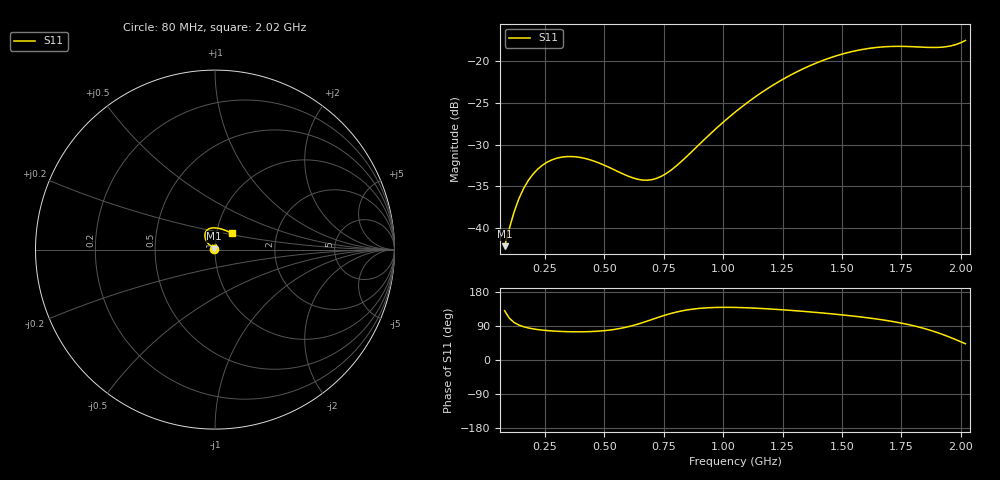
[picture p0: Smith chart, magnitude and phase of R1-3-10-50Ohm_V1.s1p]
!version-1
!date-08.2020
!Series
#	GHZ S RI R 50.0
!	FREQ.GHZ	S11RE	S11IM
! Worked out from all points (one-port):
!   98 points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, 80 MHz to 2.02 GHz, reference 50 ohm
!   lowest |S11| = -42.1 dB at 80 MHz (marker M1), VSWR 1.02, Z = 49.5 + j0.593 ohm
!   |S11| at or under -10 dB: start of sweep to end of sweep
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0.08  -0.00505 0.00599
0.12  -0.00197 0.0124
0.14  -0.000589 0.015
0.16  0.000676 0.0173
0.18  0.00183 0.0192
0.22  0.0038 0.0223
0.26  0.00532 0.0243
0.3  0.00639 0.0254
0.34  0.00701 0.0259
0.38  0.00719 0.0257
0.44  0.00665 0.0247
0.58  0.00185 0.021
0.64  -0.00156 0.0196
0.7  -0.00567 0.0187
0.72  -0.00717 0.0185
0.76  -0.0104 0.0185
0.82  -0.0155 0.0193
0.96  -0.0286 0.0253
1.06  -0.0379 0.0335
1.18  -0.0477 0.0472
1.3  -0.0544 0.0644
1.42  -0.056 0.0832
1.54  -0.0504 0.1012
1.66  -0.035 0.1152
1.78  -0.00737 0.1212
1.92  0.0443 0.1118
1.98  0.0741 0.1004
2.02  0.0967 0.0898
